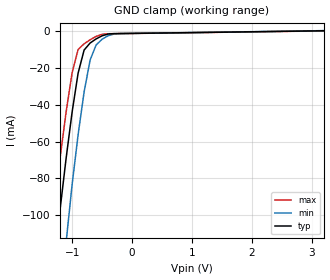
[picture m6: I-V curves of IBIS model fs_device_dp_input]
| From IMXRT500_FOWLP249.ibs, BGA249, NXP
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[Model] fs_device_dp_input
|   Model fs_device_dp_input
| Library cells for typ/min/max conditions are connected as defined below:
|  pad_usbdp - External Pad
|  d_dmpulldn - gnda
|  d_dppulldn - gnda
|  d_sw1_neg - gnda
|  d_sw1_pos - vddd
|  d_sw2_neg - gnda
|  d_sw2_pos - gnda
|  gnda - gnda
|  pad_usb_vss - pad_usb_vss
|  usb2_reg_tx_fs_hiz - vddd
|  usb2_reg_tx_hs_term - gnda
|  usb2_reg_tx_hs_xcvr - gnda
|  usb2_reg_tx_ls_en - gnda
|  usbphy_d2a_txhsactive - gnda
|  vddb - vddb
|  vddd - vddd
| All other pins connected to ground
Model_type Input
Vinl =   0.800V
Vinh =   2.000V
C_comp   2.8431pF   2.6338pF   3.0727pF
[Temperature Range]   27.0000   0.1250k   -40.0000
[Voltage Range]   3.1500V   3.0000V   3.3000V
[GND_clamp]
|Voltage   I(typ)   I(min)   I(max)
-3.3V     -1.772A    -1.863A    -1.687A
-1.4V     -159.2mA   -243.7mA   -124.9mA
-1.3V     -126.2mA   -193.7mA   -95.62mA
-1.2V     -96.43mA   -151mA     -68.52mA
-1.1V     -68.93mA   -114.4mA   -43.89mA
-1V       -43.96mA   -83.2mA    -22.65mA
-900mV    -22.89mA   -56.23mA   -10.14mA
-800mV    -10.42mA   -33.09mA   -7.028mA
-700mV    -6.621mA   -15.84mA   -4.859mA
-600mV    -4.391mA   -7.726mA   -3.047mA
-200mV    -1.483mA   -1.491mA   -1.509mA
3.2V      23.03uA    130.6uA    -44.12uA
